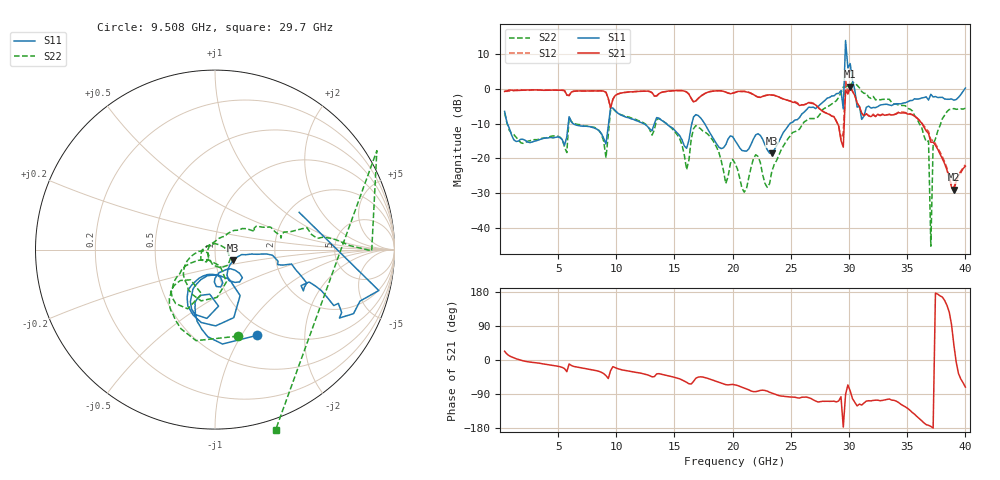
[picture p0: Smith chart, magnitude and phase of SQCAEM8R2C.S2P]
! Network Analyzer HP8722ES.07.66: Jul 25, 2000 Serial No. US39175408
! 26 Oct 2004  15:53:21
! Frequency  S11  S21  S12  S22
# HZ  S  DB R  50
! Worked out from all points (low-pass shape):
!   201 points, 400 MHz to 40 GHz, reference 50 ohm
!   highest |S21| = 0.58 dB at 30.1 GHz (marker M1); lowest = -29.0 dB at 39.01 GHz (marker M2)
!   |S21| within 3 dB of the highest: start of sweep to 9.271 GHz; 9.813 GHz to 16.38 GHz (6.568 GHz wide, 50.2 % of centre)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
!   lowest |S11| = -18.6 dB at 23.37 GHz (marker M3), VSWR 1.27, Z = 60.9 - j7.3 ohm
!   |S11| at or under -10 dB: 639.6 MHz to 5.876 GHz (5.237 GHz wide, 161 % of centre); 6.29 GHz to 9.332 GHz (3.042 GHz wide, 38.9 % of centre); 17.59 GHz to 24.92 GHz (7.331 GHz wide, 34.5 % of centre)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
!   |S22| runs from -45.2 to 1.8 dB; largest |S21 - S12| = 0.61
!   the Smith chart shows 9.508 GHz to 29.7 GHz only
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4e8  -6.51 -69.8  -0.77 23.0  -0.71 26.0  -6.91 -63.2
7.132e9  -10.76 -101.2  -0.65 -21.5  -0.66 -21.6  -10.56 -121.7
1.3666e10  -8.44 -107.2  -1.42 -36.0  -1.39 -35.8  -8.59 -126.0
1.6042e10  -17.09 -85.8  -0.94 -58.8  -0.92 -58.7  -23.20 -126.2
2.02e10  -14.85 -91.1  -1.11 -65.7  -1.02 -64.7  -21.41 -159.2
2.3368e10  -18.58 -30.1  -1.80 -87.2  -1.80 -86.3  -23.68 71.3
2.6932e10  -5.30 -25.0  -4.26 -105.2  -4.17 -104.8  -8.55 9.9
2.9308e10  -0.53 -14.0  -14.81 -97.1  -14.48 -95.4  -1.18 -0.4
2.9506e10  -5.80 23.9  -16.76 -177.1  -12.55 -141.9  0.48 31.4
2.9704e10  13.86 -61.4  -0.44 -90.5  2.44 -65.9  0.51 -71.4
2.9902e10  5.97 -64.5  -1.50 -65.8  -1.53 -64.8  0.77 -14.7
3.01e10  7.22 -86.6  0.58 -81.6  0.66 -80.8  0.99 -22.2
3.0496e10  -0.37 -89.8  -1.93 -111.7  -1.82 -110.1  1.63 -53.2
3.0694e10  -5.27 95.5  -4.04 -121.2  -4.02 -119.5  1.01 118.4
3.1288e10  -7.81 141.6  -7.74 -113.6  -7.84 -114.0  -1.32 111.5
3.1486e10  -5.32 -39.4  -7.19 -108.3  -7.18 -108.9  -1.32 -70.2
3.3466e10  -4.66 -23.0  -7.37 -102.8  -7.33 -101.8  -3.03 -70.5
3.6832e10  -3.25 -39.4  -12.81 -172.3  -12.25 -168.8  -14.96 -23.3
3.703e10  -1.58 -41.3  -15.35 -175.3  -14.64 -170.9  -45.17 -23.9
3.7228e10  -2.35 -45.2  -15.32 -179.5  -14.83 -176.3  -16.00 6.3
3.901e10  -3.26 -43.4  -28.95 39.8  -28.28 44.2  -5.68 5.8
4e10  0.21 -31.0  -22.21 -71.6  -21.82 -70.1  -5.59 -2.4
